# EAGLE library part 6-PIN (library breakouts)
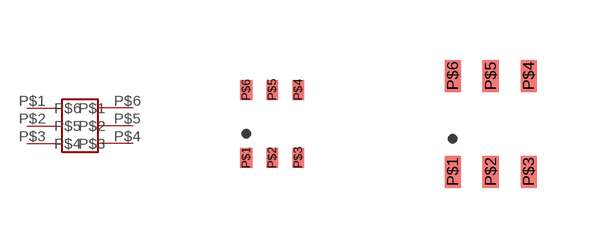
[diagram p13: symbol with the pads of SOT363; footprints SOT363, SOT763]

Designator prefix -

## 6-PINSOT363  [SOT363]
P$1  P$1
P$2  P$2
P$3  P$3
P$4  P$4
P$5  P$5
P$6  P$6

## 6-PINSOT763  [SOT763]
Pads as for SOT363

## Footprint SOT363 (pad centres in mm)
smd 0.3 x 0.5: P$1 -0.65,-0.85; P$2 0,-0.85; P$3 0.65,-0.85; P$4 0.65,0.85; P$5 0,0.85; P$6 -0.65,0.85

## Footprint SOT763 (pad centres in mm)
smd 0.4 x 0.8: P$1 -0.95,-1.2; P$2 0,-1.2; P$3 0.95,-1.2; P$4 0.95,1.2; P$5 0,1.2; P$6 -0.95,1.2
